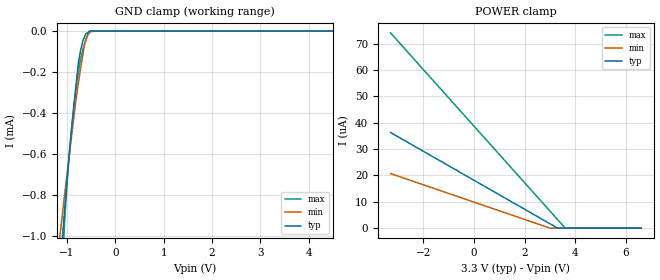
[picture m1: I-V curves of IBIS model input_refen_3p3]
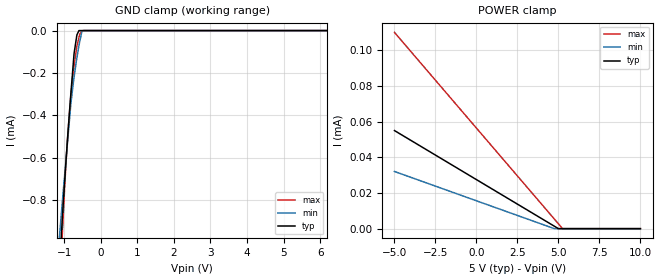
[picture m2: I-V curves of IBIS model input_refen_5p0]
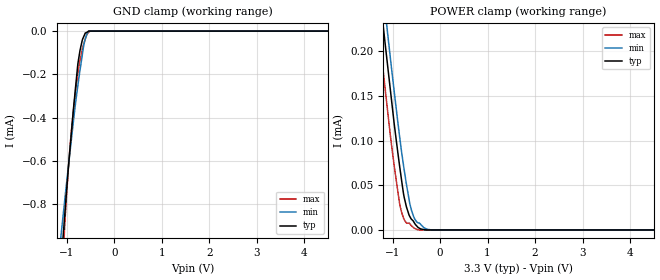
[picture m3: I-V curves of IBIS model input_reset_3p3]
|Texas Instruments Incorporated
|16-bit, 5 MSPS Delta-Sigma, Analog-to-Digital Converter
| Marketing part#   Digital Voltage Range   Package-type   #pins
| ADS1605IPAPT   2.7 to 5.25V   HTQFP   64
| ADS1605IPAPTG4   2.7 to 5.25V   HTQFP   64
| ADS1605IPAPR   2.7 to 5.25V   HTQFP   64
| ADS1605IPAPRG4   2.7 to 5.25V   HTQFP   64
[IBIS Ver]   3.2
[File name]   ads1605.ibs
|SIMDE Ver   V2.0 - 201002 - RHL4 - Build 372
[File Rev]   1.2
[Date]   09/24/2010
[Source]
|   Texas Instruments Incorporated.
|   Analog-eLab Design Center, HPA
|   12500 TI Blvd
|   Dallas, TX -75243
|   e-mail: elab_ibis@list.ti.com
| Model generated from simulations in TISPICE
[Notes]   Revision History:
|   Rev 1.0: 07/13/2010
|   - Initial version of the model
|   Rev 1.1: 07/31/2010
|   - Corrected Vinl,Vinh values
|   - Corrected volatage range for I-V tables
|   - Corrected R_pkg,L_pkg,C_pkg values
|   Rev 1.2: 09/24/2010
|   - Updated input_refen and input_pu models with the Models 2010.09.16
|   - Model generated from simulations in TISPICE
|   - Model matched to SPICE simulation
|   - Model names with a trailing 3p3 contains the model for
|   3.3V [3.0V and 3.6V]. Model names with trailing 5p0 contains
|   the model for 5.0V [4.75V and 5.25V] operation.
|   - Included new models input_pu_3p3 and input_pu_5p0
|   - C_comp although listed in numerical order of value are obtained
|   from varying PVT conditions. For PVT conditions for each specific
|   value refer the buffer description under respective [Model]. IBIS
|   model user is responsible for using appropriate C_comp to simulate
|   for Signal Integrity.
[Disclaimer]
| This model is designed as an aid for customers of Texas Instruments.
| TI and its licensors and suppliers make no warranties, either expressed
| or implied, with respect to this  model, including the warranties of
| merchantability or fitness for a particular purpose. The model is
| provided solely on an "as is" basis. The entire risk as to its quality
| and performance is with the customer.
[Copyright]
|(C) Copyright 2010 Texas Instruments Incorporated.All rights reserved.
|   ADS1605
[Component]   ADS1605
[Manufacturer]  TI
[Package]   | 64 HTQFP - PAP package
|   typ   min   max
R_pkg   0.127365   0.067657   0.170020
L_pkg   2.018606nH   1.057475nH   2.743500nH
C_pkg   0.202000pF   0.125140pF   0.402020pF
[Pin]  signal_name model_name  R_pin   L_pin   C_pin
1   AGND   GND   0.080992   1.296372nH   0.401940pF
2   AVDD   POWER   0.076992   1.225121nH   0.392300pF
3   AGND   GND   0.073902   1.170195nH   0.373140pF
4   AINN   TERM   0.071650   1.130245nH   0.359500pF
5   AINP   TERM   0.069970   1.100546nH   0.349310pF
6   AGND   GND   0.068872   1.081223nH   0.342660pF
7   AVDD   POWER   0.068165   1.068874nH   0.330150pF
8   RBIAS   TERM   0.136810   2.146100nH   0.138650pF
9   AGND   GND   0.067837   1.063300nH   0.334320pF
10   AVDD   POWER   0.067902   1.064700nH   0.337460pF
11   AGND   GND   0.067902   1.073149nH   0.339930pF
12   AVDD   POWER   0.069282   1.089672nH   0.340110pF
13   _REFEN   INPUT_REFEN 0.141430   2.230700nH   0.137900pF
14   NC   NC   0.000000   0.000000nH   0.000000pF
15   2XMODE   INPUT_REFEN 0.157540   2.519600nH   0.138910pF
16   NC   NC   0.000000   0.000000nH   0.000000pF
17   _PD   INPUT_PU   0.165610   2.665000nH   0.161790pF
18   DVDD   POWER   0.077852   1.244045nH   0.395260pF
19   DGND   GND   0.074605   1.186194nH   0.367750pF
20   _RESET   INPUT_RESET 0.153700   2.452500nH   0.153490pF
21   _CS   INPUT_RESET 0.145990   2.315100nH   0.152570pF
22   _RD   INPUT_RESET 0.140400   2.215600nH   0.144160pF
23   OTR   OUTPUT   0.137480   2.163700nH   0.137570pF
24   _DRDY   OUTPUT   0.135990   2.137300nH   0.138630pF
25   DGND   GND   0.067648   1.062500nH   0.332300pF
26   DVDD   POWER   0.067810   1.065375nH   0.324390pF
27   NC   NC   0.000000   0.000000nH   0.000000pF
28   NC   NC   0.000000   0.000000nH   0.000000pF
29   DOUT[0]   OUTPUT   0.143930   2.278400nH   0.135780pF
30   DOUT[1]   OUTPUT   0.149810   2.383100nH   0.150200pF
31   DOUT[2]   OUTPUT   0.157600   2.522000nH   0.158640pF
32   DOUT[3]   OUTPUT   0.167500   2.698800nH   0.157510pF
33   DOUT[4]   OUTPUT   0.170020   2.743500nH   0.158080pF
34   DOUT[5]   OUTPUT   0.161530   2.591100nH   0.159970pF
35   DOUT[6]   OUTPUT   0.15470   2.468700nH   0.153330pF
36   DOUT[7]   OUTPUT   0.149290   2.371700nH   0.147610pF
37   DOUT[8]   OUTPUT   0.145040   2.295400nH   0.143070pF
38   DOUT[9]   OUTPUT   0.141730   2.236100nH   0.139520pF
39   DOUT[10]   OUTPUT   0.139220   2.190900nH   0.136760pF
40   DOUT[11]   OUTPUT   0.137370   2.157700nH   0.134380pF
41   DOUT[12]   OUTPUT   0.136040   2.133600nH   0.132830pF
42   DOUT[13]   OUTPUT   0.135520   2.123900nH   0.132350pF
43   DOUT[14]   OUTPUT   0.135660   2.126000nH   0.131760pF
44   DOUT[15]   OUTPUT   0.136580   2.141900nH   0.125140pF
45   NC   NC   0.000000   0.000000nH   0.000000pF
46   NC   NC   0.000000   0.000000nH   0.000000pF
47   NC   NC   0.000000   0.000000nH   0.000000pF
48   NC   NC   0.000000   0.000000nH   0.000000pF
49   NC   NC   0.000000   0.000000nH   0.000000pF
50   NC   NC   0.000000   0.000000nH   0.000000pF
51   DGND   GND   0.072615   1.145995nH   0.349080pF
52   DVDD   POWER   0.070517   1.108571nH   0.351470pF
53   IOVDD   POWER   0.069070   1.082747nH   0.343480pF
54   DGND   GND   0.068165   1.066574nH   0.337960pF
55   AGND   GND   0.067727   1.058750nH   0.335610pF
56   CLK   INPUT_CLK   0.067657   1.057475nH   0.334710pF
57   AGND   GND   0.067997   1.063574nH   0.337020pF
58   AVDD   POWER   0.068700   1.076073nH   0.338430pF
59   VCAP   TERM   0.069132   1.083797nH   0.340780pF
60   VREFN   TERM   0.070465   1.107595nH   0.352070pF
61   VREFN   TERM   0.072150   1.137644nH   0.361260pF
62   VMID   TERM   0.074397   1.177819nH   0.374910pF
63   VREFP   TERM   0.077350   1.230645nH   0.392850pF
64   VREFP   TERM   0.081137   1.298422nH   0.402020pF
[Model selector] INPUT_REFEN
 input_refen_3p3   3.3V digital input
 input_refen_5p0   5.0V digital input
[Model selector] INPUT_RESET
 input_reset_3p3   3.3V digital input
 input_reset_5p0   5.0V digital input
[Model selector] INPUT_CLK
 input_clk_3p3   3.3V digital input
 input_clk_5p0   5.0V digital input
[Model selector] INPUT_PU
 input_pu_3p3   3.3V digital input
 input_pu_5p0   5.0V digital input
[Model selector] OUTPUT
 output_tristate_3p3  3.3V tristate output
 output_tristate_5p0  5.0V tristate output
[Model selector] TERM
 term_3-3V   3.3V nominal termination
 term_5-0V   5.0V nominal termination
[Model] term_3-3V
Model_type Terminator
C_comp  1.0e-20F  1.0e-20F 1.0e-20F
| variable   typ   min   max
[Voltage Range]   3.30000V  3.00000V  3.60000V
[POWER Clamp Reference]  3.30000V  3.00000V  3.60000V
[GND Clamp Reference]   0.00000V  0.00000V  0.00000V
|Ambient Temperature   25   85   -40
|Junction Temperature
[Temperature Range]   39   99   -40
[Model] term_5-0V
Model_type Terminator
C_comp  1.0e-20F  1.0e-20F 1.0e-20F
| variable   typ   min   max
[Voltage Range]   5.00000V  4.75000V  5.25000V
[POWER Clamp Reference]  5.00000V  4.75000V  5.25000V
[GND Clamp Reference]   0.00000V  0.00000V  0.00000V
|Ambient Temperature   25   85   -40
|Junction Temperature
[Temperature Range]   39   99   -40
| Models and submodels in the file (12): input_refen_3p3 (Input), input_refen_5p0 (Input), input_reset_3p3 (Input), input_reset_5p0 (Input), input_pu_3p3 (Input), input_pu_5p0 (Input), input_clk_3p3 (Input), input_clk_5p0 (Input), output_tristate_3p3 (3-state), output_tristate_5p0 (3-state), term_3-3V (Terminator), term_5-0V (Terminator)
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|   INPUT_REFEN 3.3V Model
[Model]   input_refen_3p3
Model_type   Input
Vinl = 0.99
Vinh = 2.31
|   typ   min   max
|   (nom PVT)   (Fast PVT)   (Slow PVT)
C_comp   6.911e-13   5.974e-13   7.264e-13
|Where nom PVT is NOM Process, 3.3V,39C
|   Fast PVT is Strong Process, 3.6V, -40C
|   Slow PVT is Weak Process, 3.0V, 99C
[Model Spec]
Vinl   0.99   0.9   1.08
Vinh   2.31   2.1   2.52
[Voltage Range]   3.3   3   3.6
|Ambient Temperature   25   85   -40
|Junction Temperature
[Temperature Range]   39   99   -40
[Power Clamp Reference]   3.3   3   3.6
[GND Clamp Reference]   0   0   0
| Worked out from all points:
|   GND clamp passes 1 mA (typ) near -1.09 V on its own axis
[GND Clamp]
|   Voltage   I(typ)   I(min)   I(max)
-3.3V     -8mA       -5.73mA    -13.12mA
-1.14V    -1.146mA   -991.1uA   -1.369mA
-1.046V   -870.9uA   -797.8uA   -929.1uA
-988.8mV  -705.3uA   -679.2uA   -721.5uA
-909.6mV  -494.3uA   -524.7uA   -491.9uA
-816mV    -273.9uA   -343.4uA   -291.6uA
-765.6mV  -161.6uA   -260.1uA   -204uA
-719.4mV  -97.46uA   -186.5uA   -140.6uA
-639mV    -30.31uA   -69.93uA   -64.47uA
-537mV    0A         -3.653uA   -9.909uA
-369.6mV  0A         0A         0A
6.6V      0A         0A         0A
[POWER Clamp]
|   Voltage   I(typ)   I(min)   I(max)
-3.3V     36.28uA    20.71uA    74.05uA
3V        1.649uA    0A         6.45uA
3.3V      0A         0A         3.231uA
3.601V    0A         0A         0A
6.6V      0A         0A         0A
|   INPUT_REFEN 5.0V Model
[Model]   input_refen_5p0
Model_type   Input
Vinl = 1.5
Vinh = 3.5
|   typ   min   max
|   (nom PVT)   (Fast PVT)   (Slow PVT)
C_comp   6.242e-13   5.411e-13   6.719e-13
|Where nom PVT is NOM Process, 5.0V,39C
|   Fast PVT is Strong Process, 5.25V, -40C
|   Slow PVT is Weak Process, 4.75V, 99C
[Model Spec]
Vinl   1.5   1.425   1.575
Vinh   3.5   3.325   3.675
[Voltage Range]   5   4.75   5.25
|Ambient Temperature   25   85   -40
|Junction Temperature
[Temperature Range]   39   99   -40
[Power Clamp Reference]   5   4.75   5.25
[GND Clamp Reference]   0   0   0
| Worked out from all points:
|   GND clamp passes 1 mA (typ) near -1.09 V on its own axis
[GND Clamp]
|   Voltage   I(typ)   I(min)   I(max)
-5V       -13.49mA   -9.526mA   -22.86mA
-1.136V   -1.14mA    -985.2uA   -1.355mA
-1.062V   -918uA     -831.4uA   -1mA
-1.05V    -880.3uA   -805.6uA   -953.9uA
-947mV    -605.4uA   -601.1uA   -614.4uA
-826.3mV  -316.3uA   -361.4uA   -323.7uA
-730mV    -107.9uA   -220.5uA   -165.6uA
-650mV    -19.27uA   -124.8uA   -70.65uA
-596.8mV  0A         -69.79uA   -32.1uA
-520.8mV  0A         -7.187uA   -1.927uA
-480mV    0A         0A         -618.5nA
10V       0A         0A         0A
[POWER Clamp]
|   Voltage   I(typ)   I(min)   I(max)
-5V       54.97uA    32.05uA    110uA
4.752V    1.365uA    0A         5.379uA
5V        0A         0A         2.716uA
5.253V    0A         0A         0A
10V       0A         0A         0A
|   INPUT_RESET 3.3V Model
[Model]   input_reset_3p3
Model_type   Input
Vinl = 0.99
Vinh = 2.31
|   typ   min   max
|   (nom PVT)   (Fast PVT)   (Slow PVT)
C_comp   7.724e-13   7.499e-13   7.980e-13
|Where nom PVT is NOM Process, 3.3V,39C
|   Fast PVT is Strong Process, 3.6V, -40C
|   Slow PVT is Weak Process, 3.0V, 99C
[Model Spec]
Vinl   0.99   0.9   1.08
Vinh   2.31   2.1   2.52
[Voltage Range]   3.3   3   3.6
|Ambient Temperature   25   85   -40
|Junction Temperature
[Temperature Range]   39   99   -40
[Power Clamp Reference]   3.3   3   3.6
[GND Clamp Reference]   0   0   0
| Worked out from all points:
|   GND clamp passes 1 mA (typ) near -1.09 V on its own axis
[GND Clamp]
|   Voltage   I(typ)   I(min)   I(max)
-3.3V     -7.999mA   -5.729mA   -13.84mA
-1.136V   -1.131mA   -980.6uA   -1.346mA
-1.043V   -855.6uA   -785.4uA   -904.7uA
-970.8mV  -648uA     -639.3uA   -654.9uA
-906mV    -482.7uA   -510.1uA   -474.5uA
-816mV    -266.2uA   -337.7uA   -284.4uA
-765.6mV  -152.7uA   -253.1uA   -197.3uA
-719.4mV  -89.13uA   -180.5uA   -136.3uA
-642mV    -25.67uA   -67.07uA   -61.07uA
-582mV    -6.335uA   -17.39uA   -20.43uA
-537mV    0A         0A         -5.427uA
6.6V      0A         0A         0A
[POWER Clamp]
|   Voltage   I(typ)   I(min)   I(max)
-3.3V     1.305mA    1.336mA    1.261mA
-1.299V   279.1uA    315.2uA    228.9uA
-1.234V   246.9uA    283.4uA    196.3uA
-1.165V   213.3uA    249.9uA    162.9uA
-1.146V   204.3uA    240.7uA    153.9uA
-1.046V   157.5uA    193.2uA    106.4uA
-841.2mV  68.01uA    100.7uA    26.91uA
-706.2mV  25.71uA    51.02uA    7.773uA
-597mV    11.79uA    21.46uA    4.584uA
-492mV    4.588uA    9.139uA    661.2nA
-171.6mV  0A         0A         0A
6.6V      0A         0A         0A
